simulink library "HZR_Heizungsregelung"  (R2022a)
settings: Solver=VariableStepAuto  StartTime=0.0  StopTime=10.0  RelTol=1e-3
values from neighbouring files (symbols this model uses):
  PAR_HZR_Beginn_Nachtzeit = 22    [parameter_HZR.m]
  PAR_HZR_Beginn_Tageszeit = 5    [parameter_HZR.m]
  PAR_HZR_D = 0    [parameter_HZR.m]
  PAR_HZR_Heizleistung_Warmwasser = 200    [parameter_HZR.m]
  PAR_HZR_I = 0.001    [parameter_HZR.m]
  PAR_HZR_Max_Heizung = 30    [parameter_HZR.m]
  PAR_HZR_Min_Klima = 18    [parameter_HZR.m]
  PAR_HZR_Minimaltemperatur = 10    [parameter_HZR.m]
  PAR_HZR_P = 3000    [parameter_HZR.m]
  PAR_HZR_Solltemperatur_Nacht = 15    [parameter_HZR.m]
  PAR_HZR_Solltemperatur_Tag = 20    [parameter_HZR.m]
  PAR_HZR_Wassertemp_Hysterese = 5    [parameter_HZR.m]
  PAR_HZR_Wassertemp_Soll = 70    [parameter_HZR.m]
  PAR_HZT_MaxLeistung_Heizung = 10000    [parameter_HZT.m]
  PAR_HZT_MinLeistung_Klima = -10000    [parameter_HZT.m]

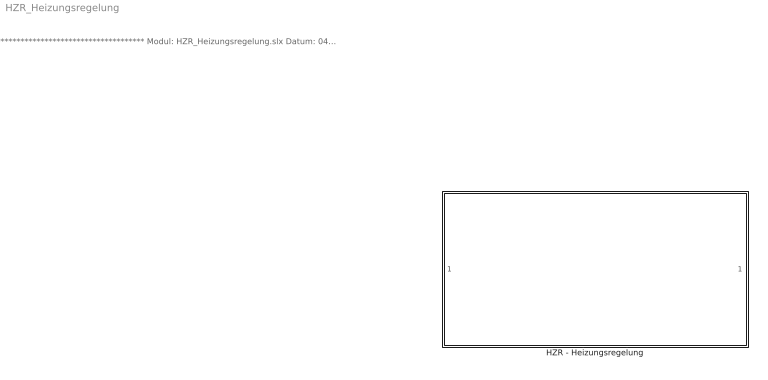
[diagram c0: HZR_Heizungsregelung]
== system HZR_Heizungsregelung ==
  note: ************************************* Modul: HZR_Heizungsregelung.slx Datum: 04. Juli 2023 Implementierung: MATLAB R2022a Toolbox: - Autor: Betten Nils, Pichmann Florian Bemerkung: Letzte Aenderung : 04. Juli 2023 *************************************
  HZR - Heizungsregelung : Subsystem

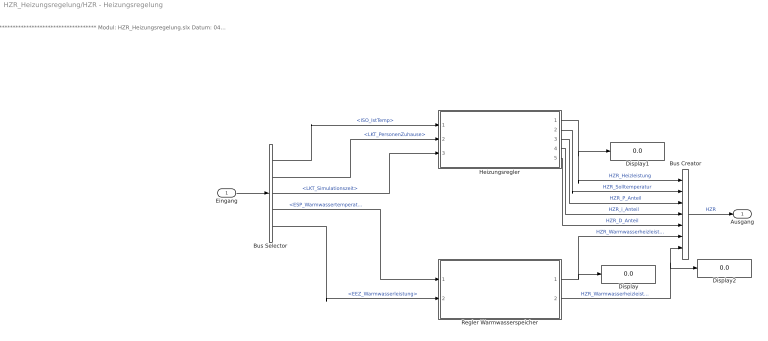
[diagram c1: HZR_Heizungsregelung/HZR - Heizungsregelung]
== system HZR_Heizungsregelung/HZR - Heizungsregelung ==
  note: ************************************* Modul: HZR_Heizungsregelung.slx Datum: 04. Juli 2023 Implementierung: MATLAB R2022a Toolbox: - Autor: Betten Nils, Pichmann Florian Bemerkung: Letzte Aenderung : 04. Juli 2023 *************************************
  Eingang : Inport
  Bus Creator : BusCreator  Inputs=7
  Bus Selector : BusSelector  OutputSignals=signal6.ISO_IstTemp,LKT.LKT_PersonenZuhause,LKT.LKT_Simulationszeit,ESP_Warmwassertemperatur,EEZ.EEZ_Warmwasserleistung
  Display : Display
  Display1 : Display
  Display2 : Display
  Heizungsregler : Subsystem
  Regler Warmwasserspeicher : Subsystem
  Ausgang : Outport
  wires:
  Bus Selector/1 -> Heizungsregler/1(ISO_Isttemperatur_Haus)  "<ISO_IstTemp>"
  Bus Selector/2 -> Heizungsregler/2(LKT_aktuellerStatus)  "<LKT_PersonenZuhause>"
  Heizungsregler/1(HZR_Heizleistung) -> Display1/1, Bus Creator/1  "HZR_Heizleistung"
  Regler Warmwasserspeicher/1(HZR_Warmwasserheizleistung) -> Bus Creator/6, Display/1  "HZR_Warmwasserheizleistung"
  Bus Creator/1 -> Ausgang/1  "HZR"
  Eingang/1 -> Bus Selector/1
  Bus Selector/3 -> Heizungsregler/3(LKT_Simulationszeit)  "<LKT_Simulationszeit>"
  Bus Selector/4 -> Regler Warmwasserspeicher/1(ESP_Warmwassertemperatur)  "<ESP_Warmwassertemperatur>"
  Bus Selector/5 -> Regler Warmwasserspeicher/2(EEZ_Warmwasserleistung)  "<EEZ_Warmwasserleistung>"
  Regler Warmwasserspeicher/2(HZR_Warmwasserheizleistung_Waermepumpe) -> Display2/1, Bus Creator/7  "HZR_Warmwasserheizleistung_Waermepumpe"
  Heizungsregler/2(HZR_Solltemperatur) -> Bus Creator/2  "HZR_Solltemperatur"
  Heizungsregler/3(HZR_Heizungsregler_P_Anteil) -> Bus Creator/3  "HZR_P_Anteil"
  Heizungsregler/4(HZR_Heizungsregler_i_Anteil) -> Bus Creator/4  "HZR_i_Anteil"
  Heizungsregler/5(HZR_Heizungsregler_D_Anteil) -> Bus Creator/5  "HZR_D_Anteil"

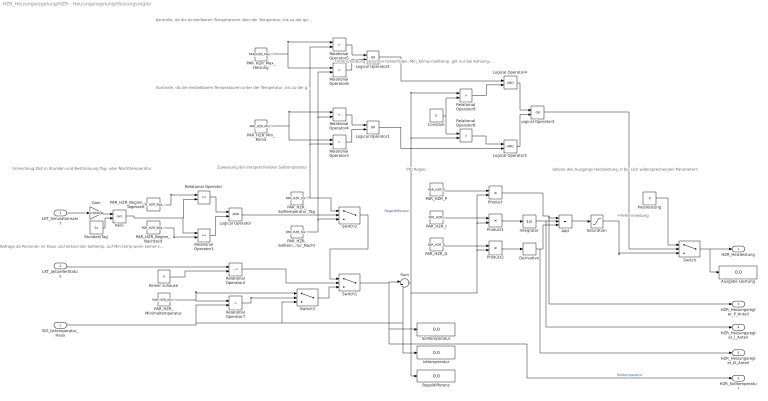
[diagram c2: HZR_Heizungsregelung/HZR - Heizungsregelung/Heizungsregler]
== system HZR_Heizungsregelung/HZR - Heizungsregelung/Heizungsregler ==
  note: Unterscheidung zwischen Fehlerfällen: Min_Klima>Solltemp. gilt nur bei Kühlung; Max_Heizung<Solltemp. nur bei Heizung
  note: Setzen des Ausgangs Heizleistung, 0 bei sich widersprechenden Parametern
  note: PID Regler
  note: +Fehlermeldung
  note: Kontrolle, ob die einstellbaren Temperaturen über der Temperatur, bis zu der geheizt wird, liegen
  note: Kontrolle, ob die einstellbaren Temperaturen unter der Temperatur, bis zu der gekühlt wird, liegen
  note: Zuweisung der entsprechenden Solltemperatur
  note: Abfrage ob Personen im Haus und Setzen der Solltemp. auf Min.temp wenn keiner zuhause ist und die Isttemp. zu gering ist
  note: Umrechnug Zeit in Stunden und Bestimmung Tag- oder Nachttemperatur
  ISO_Isttemperatur_Haus : Inport
  LKT_aktuellerStatus : Inport  Port=2
  LKT_Simulationszeit : Inport  Port=3
  Add : Sum  Inputs=+++
  Ausgabe Leistung : Display
  Constant : Constant  Value=0
  Derivative : Derivative
  Gain : Gain  Gain=1/3600
  Heizleistung : Constant  Value=0
  Integrator : Integrator
  Isttemperatur : Display
  Keiner zuhause : Constant  Value=0
  Logical Operator : Logic  AllPortsSameDT=off  OutDataTypeStr=boolean
  Logical Operator1 : Logic  Operator=OR  AllPortsSameDT=off  OutDataTypeStr=boolean
  Logical Operator2 : Logic  Operator=OR  AllPortsSameDT=off  OutDataTypeStr=boolean
  Logical Operator3 : Logic  Operator=OR  AllPortsSameDT=off  OutDataTypeStr=boolean
  Logical Operator4 : Logic  AllPortsSameDT=off  OutDataTypeStr=boolean
  Logical Operator5 : Logic  AllPortsSameDT=off  OutDataTypeStr=boolean
  PAR_HZR_Beginn_Nachtzeit : Constant  Value=PAR_HZR_Beginn_Nachtzeit
  PAR_HZR_Beginn_Tageszeit : Constant  Value=PAR_HZR_Beginn_Tageszeit
  PAR_HZR_D : Constant  Value=PAR_HZR_D
  PAR_HZR_I : Constant  Value=PAR_HZR_I
  PAR_HZR_Max_Heizung : Constant  Value=PAR_HZR_Max_Heizung
  PAR_HZR_Min_Klima : Constant  Value=PAR_HZR_Min_Klima
  PAR_HZR_Minimaltemperatur : Constant  Value=PAR_HZR_Minimaltemperatur
  PAR_HZR_P : Constant  Value=PAR_HZR_P
  PAR_HZR_Solltemperatur_Nacht : Constant  Value=PAR_HZR_Solltemperatur_Nacht
  PAR_HZR_Solltemperatur_Tag : Constant  Value=PAR_HZR_Solltemperatur_Tag
  Product : Product
  Product1 : Product
  Product2 : Product
  Regeldifferenz : Display
  Relational Operator : RelationalOperator  Operator=<=  OutDataTypeStr=boolean  RndMeth=Simplest
  Relational Operator1 : RelationalOperator  Operator=<=  OutDataTypeStr=boolean  RndMeth=Simplest
  Relational Operator2 : RelationalOperator  Operator=~=  OutDataTypeStr=boolean  RndMeth=Simplest
  Relational Operator{3..4,7..9} (5 alike) : RelationalOperator  Operator=>  OutDataTypeStr=boolean  RndMeth=Simplest
  Relational Operator5 : RelationalOperator  Operator=<  OutDataTypeStr=boolean  RndMeth=Simplest
  Relational Operator6 : RelationalOperator  Operator=<  OutDataTypeStr=boolean  RndMeth=Simplest
  Rem : Math  Operator=rem
  Saturation : Saturate  UpperLimit=PAR_HZT_MaxLeistung_Heizung  LowerLimit=PAR_HZT_MinLeistung_Klima
  Solltemperatur : Display
  Stunden/Tag : Constant  Value=24
  Sum : Sum  Inputs=|+-
  Switch{,1..3} (4 alike) : Switch  Criteria=u2 > Threshold
  HZR_Heizleistung : Outport
  HZR_Solltemperatur : Outport  Port=2
  HZR_Heizungsregler_P_Anteil : Outport  Port=3
  HZR_Heizungsregler_i_Anteil : Outport  Port=4
  HZR_Heizungsregler_D_Anteil : Outport  Port=5
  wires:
  ISO_Isttemperatur_Haus/1 -> Isttemperatur/1, Sum/2, Switch3/3, Relational Operator7/2
  Switch/1 -> HZR_Heizleistung/1, Ausgabe Leistung/1
  PAR_HZR_Beginn_Tageszeit/1 -> Relational Operator/1
  LKT_Simulationszeit/1 -> Gain/1
  Relational Operator/1 -> Logical Operator/1
  PAR_HZR_Beginn_Nachtzeit/1 -> Relational Operator1/2
  Relational Operator1/1 -> Logical Operator/2
  Logical Operator/1 -> Switch2/2
  PAR_HZR_Solltemperatur_Nacht/1 -> Relational Operator6/2, Relational Operator4/2, Switch2/3
  PAR_HZR_Solltemperatur_Tag/1 -> Relational Operator5/2, Relational Operator3/2, Switch2/1
  Switch2/1 -> Switch1/1
  PAR_HZR_Minimaltemperatur/1 -> Switch3/1, Relational Operator7/1
  PAR_HZR_Min_Klima/1 -> Relational Operator3/1, Relational Operator4/1
  Relational Operator4/1 -> Logical Operator1/1
  Relational Operator3/1 -> Logical Operator1/2
  PAR_HZR_Max_Heizung/1 -> Relational Operator6/1, Relational Operator5/1
  Relational Operator5/1 -> Logical Operator2/1
  Relational Operator6/1 -> Logical Operator2/2
  Logical Operator3/1 -> Switch/2
  Switch1/1 -> HZR_Solltemperatur/1, Solltemperatur/1, Sum/1  "Solltemperatur"
  PAR_HZR_D/1 -> Product2/1
  PAR_HZR_I/1 -> Product1/1
  PAR_HZR_P/1 -> Product/1
  Product1/1 -> Integrator/1
  Product2/1 -> Derivative/1
  Integrator/1 -> HZR_Heizungsregler_i_Anteil/1, Add/2
  Product/1 -> HZR_Heizungsregler_P_Anteil/1, Add/1
  Derivative/1 -> HZR_Heizungsregler_D_Anteil/1, Add/3
  Add/1 -> Saturation/1
  Saturation/1 -> Switch/3
  Heizleistung/1 -> Switch/1
  LKT_aktuellerStatus/1 -> Relational Operator2/1
  Keiner zuhause/1 -> Relational Operator2/2
  Relational Operator2/1 -> Switch1/2
  Relational Operator7/1 -> Switch3/2
  Switch3/1 -> Switch1/3
  Constant/1 -> Relational Operator9/2, Relational Operator8/1
  Relational Operator9/1 -> Logical Operator4/2
  Relational Operator8/1 -> Logical Operator5/1
  Logical Operator1/1 -> Logical Operator5/2
  Logical Operator2/1 -> Logical Operator4/1
  Logical Operator4/1 -> Logical Operator3/1
  Logical Operator5/1 -> Logical Operator3/2
  Sum/1 -> Product2/2, Product1/2, Product/2, Regeldifferenz/1, Relational Operator9/1, Relational Operator8/2  "Regeldifferenz"
  Gain/1 -> Rem/1
  Rem/1 -> Relational Operator1/1, Relational Operator/2
  Stunden/Tag/1 -> Rem/2

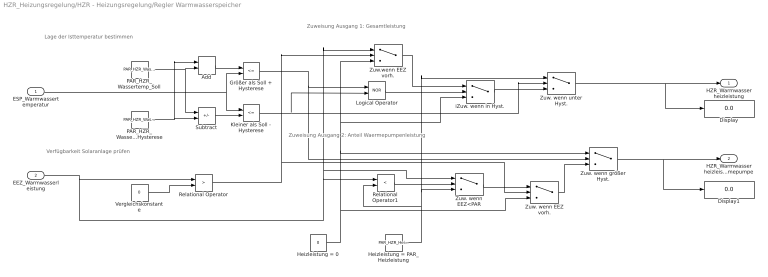
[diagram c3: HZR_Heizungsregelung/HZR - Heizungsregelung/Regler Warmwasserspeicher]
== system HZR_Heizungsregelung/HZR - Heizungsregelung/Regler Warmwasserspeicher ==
  note: Zuweisung Ausgang 2: Anteil Waermepumpenleistung
  note: Verfügbarkeit Solaranlage prüfen
  note: Zuweisung Ausgang 1: Gesamtleistung
  note: Lage der Isttemperatur bestimmen
  ESP_Warmwassertemperatur : Inport
  EEZ_Warmwasserleistung : Inport  Port=2
  Add : Sum
  Display : Display
  Display1 : Display
  Größer als Soll + Hysterese : RelationalOperator  Operator=<=  OutDataTypeStr=boolean  RndMeth=Simplest
  Heizleistung = 0 : Constant  Value=0
  Heizleistung = PAR_Heizleistung : Constant  Value=PAR_HZR_Heizleistung_Warmwasser
  Kleiner als Soll - Hysterese : RelationalOperator  Operator=<=  OutDataTypeStr=boolean  RndMeth=Simplest
  Logical Operator : Logic  Operator=NOR  AllPortsSameDT=off  OutDataTypeStr=boolean
  PAR_HZR_Wassertemp_Hysterese : Constant  Value=PAR_HZR_Wassertemp_Hysterese
  PAR_HZR_Wassertemp_Soll : Constant  Value=PAR_HZR_Wassertemp_Soll
  Relational Operator : RelationalOperator  Operator=>  OutDataTypeStr=boolean  RndMeth=Simplest
  Relational Operator1 : RelationalOperator  Operator=<  OutDataTypeStr=boolean  RndMeth=Simplest
  Subtract : Sum  Inputs=+-
  Vergleichskonstante : Constant  Value=0
  Zuw. wenn EEZ vorh. : Switch  Criteria=u2 > Threshold
  Zuw. wenn EEZ<PAR : Switch  Criteria=u2 > Threshold
  Zuw. wenn größer Hyst. : Switch  Criteria=u2 > Threshold
  Zuw. wenn unter Hyst. : Switch  Criteria=u2 > Threshold
  Zuw.wenn EEZ vorh. : Switch  Criteria=u2 > Threshold
  iZuw. wenn in Hyst. : Switch  Criteria=u2 > Threshold
  HZR_Warmwasserheizleistung : Outport
  HZR_Warmwasserheizleistung_Waermepumpe : Outport  Port=2
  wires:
  Zuw. wenn EEZ vorh./1 -> Zuw. wenn größer Hyst./3
  Zuw. wenn EEZ<PAR/1 -> Zuw. wenn EEZ vorh./1
  Größer als Soll + Hysterese/1 -> Zuw. wenn größer Hyst./2, Logical Operator/1
  Zuw. wenn größer Hyst./1 -> Display1/1, HZR_Warmwasserheizleistung_Waermepumpe/1
  Heizleistung = 0/1 -> Zuw.wenn EEZ vorh./3, iZuw. wenn in Hyst./3, Zuw. wenn größer Hyst./1, Zuw. wenn EEZ vorh./3
  Relational Operator/1 -> Zuw.wenn EEZ vorh./2, Zuw. wenn EEZ vorh./2
  Kleiner als Soll - Hysterese/1 -> Zuw. wenn unter Hyst./2, Logical Operator/2
  ESP_Warmwassertemperatur/1 -> Kleiner als Soll - Hysterese/1, Größer als Soll + Hysterese/2
  EEZ_Warmwasserleistung/1 -> Zuw.wenn EEZ vorh./1, Zuw. wenn EEZ<PAR/1, Relational Operator1/1, Relational Operator/1
  Zuw. wenn unter Hyst./1 -> HZR_Warmwasserheizleistung/1, Display/1
  Zuw.wenn EEZ vorh./1 -> iZuw. wenn in Hyst./1
  Logical Operator/1 -> iZuw. wenn in Hyst./2
  PAR_HZR_Wassertemp_Hysterese/1 -> Add/1, Subtract/2
  Relational Operator1/1 -> Zuw. wenn EEZ<PAR/2
  PAR_HZR_Wassertemp_Soll/1 -> Subtract/1, Add/2
  Add/1 -> Größer als Soll + Hysterese/1
  Subtract/1 -> Kleiner als Soll - Hysterese/2
  Vergleichskonstante/1 -> Relational Operator/2
  iZuw. wenn in Hyst./1 -> Zuw. wenn unter Hyst./3
  Heizleistung = PAR_Heizleistung/1 -> Relational Operator1/2, Zuw. wenn unter Hyst./1, Zuw. wenn EEZ<PAR/3
